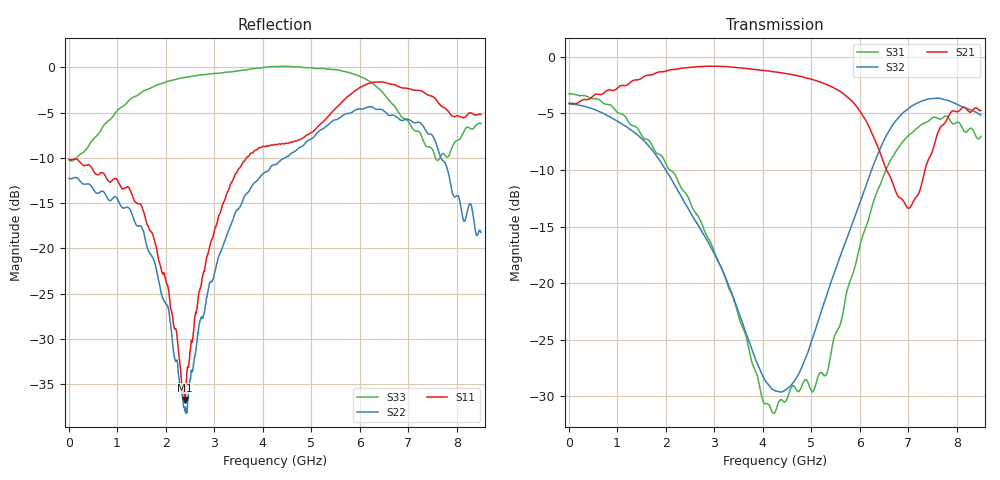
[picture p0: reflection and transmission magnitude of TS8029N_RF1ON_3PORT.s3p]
!Created with skrf (http://scikit-rf.org).
# GHz S RI R 50.0
!freq ReS11 ImS11 ReS12 ImS12 ReS13 ImS13
! ReS21 ImS21 ReS22 ImS22 ReS23 ImS23
! ReS31 ImS31 ReS32 ImS32 ReS33 ImS33
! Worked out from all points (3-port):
!   1601 points, 10 MHz to 8.5 GHz, reference 50 ohm
!   strongest paths, dB at 10 MHz, 2.132 GHz, 4.255 GHz, 6.378 GHz, 8.5 GHz:
!     S21: -4.1, -1.1, -1.3, -8.0, -4.8
!     S32: -4.2, -10.9, -29.5, -8.6, -5.2
!     S31: -3.3, -10.1, -31.4, -11.7, -7.0
!   lowest |S11| = -36.8 dB at 2.393 GHz (marker M1), VSWR 1.03, Z = 48.6 + j0.00112 ohm
!   |S11| at or under -10 dB: start of sweep to 3.663 GHz
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0.01  -0.3108 0.00382  0.6233 4.17e-05  0.6862 -0.00671
      0.6231 2.17e-05  -0.2439 0.00284  0.619 -0.0072
      0.686 -0.0068  0.6191 -0.00728  -0.3068 0.0106
1.002269  -0.1684 0.1689  0.7185 -0.1027  0.3306 -0.462
          0.7185 -0.1029  -0.09 0.165  0.266 -0.4461
          0.3304 -0.4619  0.2666 -0.4463  0.3286 0.474
1.761062  -0.0471 0.1027  0.7652 -0.3465  -0.00953 -0.3894
          0.765 -0.3464  0.0437 0.0737  -0.0948 -0.3651
          -0.00936 -0.3896  -0.0952 -0.3654  0.7862 0.0209
2.392506  -0.0145 1.15e-05  0.6747 -0.5855  -0.1184 -0.2227
          0.6744 -0.5855  0.00542 -0.0116  -0.1678 -0.1528
          -0.1181 -0.2225  -0.1674 -0.1527  0.7327 -0.4873
3.204362  -0.133 -0.1231  0.4119 -0.8064  -0.0916 -0.06
          0.4125 -0.8059  -0.1025 -0.0318  -0.1099 -0.000579
          -0.0913 -0.06  -0.1101 -0.000477  0.1502 -0.9249
4.255  -0.3369 -0.1639  -0.0346 -0.8563  -0.00936 -0.0253
       -0.0349 -0.8555  -0.2878 0.0344  7.19e-05 0.0335
       -0.00944 -0.0252  5.2e-05 0.0335  -0.5653 -0.8373
5.2738  -0.5089 0.0193  -0.3933 -0.6516  -0.0389 0.00375
        -0.3929 -0.6524  -0.2119 0.4121  0.0435 0.0706
        -0.0389 0.00369  0.0435 0.0705  -0.9843 -0.0292
6.409338  -0.5401 0.6314  -0.3447 -0.1709  0.1587 0.2164
          -0.3442 -0.1713  0.1653 0.5621  0.3764 0.0886
          0.1587 0.2164  0.3766 0.0881  -0.4374 0.6173
7.52365  0.0988 0.6788  -0.0706 -0.3906  0.394 -0.3692
         -0.0705 -0.391  0.4094 -0.0387  0.1356 -0.6406
         0.3953 -0.3689  0.1361 -0.6399  0.1769 0.2921
8.5  0.1654 0.5233  -0.3742 -0.4412  -0.1134 -0.4299
     -0.3747 -0.4408  0.1211 0.0186  -0.4228 -0.3543
     -0.1137 -0.4298  -0.4225 -0.3551  0.4049 0.2731
